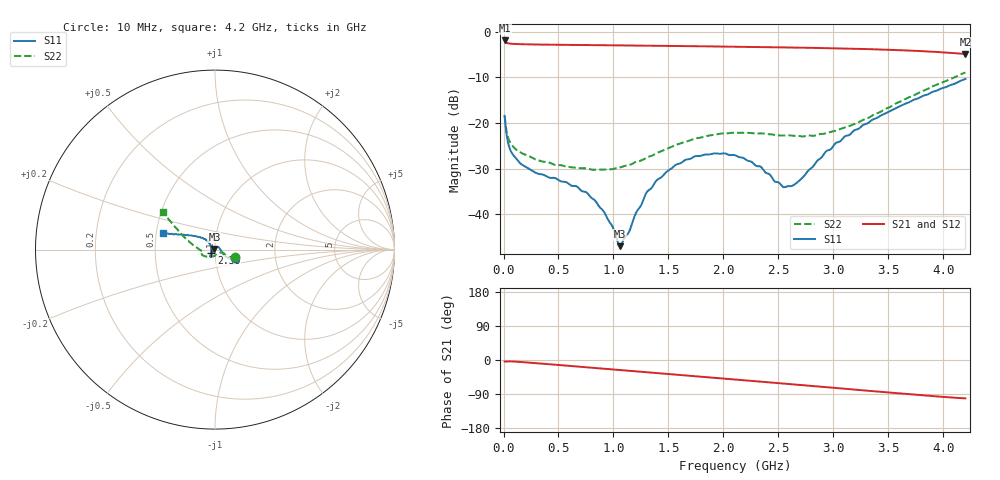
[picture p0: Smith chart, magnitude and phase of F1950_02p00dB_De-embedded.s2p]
! Integrated Device Technology
! Corporate Headquarters
! 6024 Silver Creek Valley Road
! San Jose, CA 95138  USA
! Phone:  1-408-284-8200
! Toll Free:  1-800-223-1366
! Webpage:  http://www.idt.com/
! Timing and RF Division
! 515 Groton Road, Suite 102
! Westford, MA 01886-6024
! Device:  F1950
! Description: 7-bit 0.25 dB Digital Step Attenuator
! Frequency:  150.0 -  4000.00 MHz
! Package:  4x4 mm Thin QFN Plastic Package: 24 pin
! Ports:  2 RF, 12 DC
!  Pin  1  = D0
!  Pin  2  = VDD
!  Pin  3  = Vmode
!  Pin  4  = GND
!  Pin  5  = RF1  =  Port 1
!  Pin  6  = GND
!  Pin  7  = GND
!  Pin  8  = GND
!  Pin  9  = GND
!  Pin 10  = GND
!  Pin 11  = GND
!  Pin 12  = GND
!  Pin 13  = GND
!  Pin 14  = RF2  =  Port 2
!  Pin 15  = GND
!  Pin 16  = LE
!  Pin 17  = CLK
!  Pin 18  = DATE
!  Pin 19  = D6
!  Pin 20  = D5
!  Pin 21  = D4
!  Pin 22  = D3
!  Pin 23  = D2
!  Pin 24  = D1
! State:  8
! Atten State:  2.00 dB
! Voltage:  +5.00 Volts
! Current:  Not Measured mA
! Data:  The device was measured on a the F195X evaluation board which has
!  individual transmission lines to the RF pins.  Data was collected
!  using a calibrated network analyzer.  The evaluation board was
!  de-embedded using a TRL calibration technique.
!  The reference plane is the edge of the package pin.
! Misc:  Board 2019
!  Action Tracker AT0250
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# GHz S dB R 50
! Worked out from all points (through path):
!   420 points, 10 MHz to 4.2 GHz, reference 50 ohm
!   highest |S21| = -1.93 dB at 10 MHz (marker M1); lowest = -4.9 dB at 4.2 GHz (marker M2)
!   group delay of S21, straight-line fit = 66.8 ps
!   lowest |S11| = -47.0 dB at 1.06 GHz (marker M3), VSWR 1.01, Z = 49.7 + j0.33 ohm
!   |S11| at or under -10 dB: start of sweep to end of sweep
!   |S22| runs from -30.2 to -8.9 dB; largest |S21 - S12| = 0.00089
!   S11 on the Smith chart (normalised r, x): 10 MHz: 1.24, -0.12; 2.39 GHz: 0.96, -0.04; 4.2 GHz: 0.54, +0.11
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0.01  -18.44 -22.7  -1.93 -3.8  -1.93 -3.8  -18.41 -20.7
0.06  -25.81 -27.8  -2.62 -3.6  -2.62 -3.6  -24.21 -26.0
0.16  -28.98 -12.3  -2.75 -5.3  -2.74 -5.3  -26.51 -22.1
0.3  -30.96 7.5  -2.82 -8.5  -2.82 -8.5  -28.06 -22.9
0.47  -32.05 28.0  -2.87 -12.4  -2.87 -12.4  -29.18 -25.8
0.71  -34.86 51.8  -2.93 -18.1  -2.92 -18.1  -29.89 -39.5
0.82  -36.71 61.0  -2.95 -20.8  -2.95 -20.8  -30.23 -49.6
0.91  -39.31 74.8  -2.97 -22.9  -2.97 -22.9  -30.20 -60.0
1.06  -46.95 132.3  -3.01 -26.5  -3.01 -26.5  -29.71 -81.7
1.14  -43.88 -170.3  -3.03 -28.4  -3.02 -28.4  -29.18 -92.7
1.3  -35.22 -139.2  -3.06 -32.2  -3.06 -32.2  -27.61 -112.8
1.41  -32.22 -132.3  -3.09 -34.9  -3.09 -34.9  -26.41 -123.9
1.56  -29.24 -128.3  -3.14 -38.5  -3.13 -38.5  -24.86 -135.6
1.74  -27.30 -124.8  -3.19 -42.8  -3.19 -42.8  -23.41 -146.2
2.11  -27.09 -123.7  -3.31 -51.7  -3.30 -51.7  -22.16 -159.9
2.39  -30.95 -137.7  -3.40 -58.4  -3.40 -58.4  -22.40 -165.2
2.57  -33.94 -172.2  -3.46 -62.7  -3.45 -62.7  -22.69 -168.7
2.66  -33.19 161.3  -3.49 -64.9  -3.48 -64.9  -22.78 -169.9
2.81  -29.64 136.9  -3.55 -68.6  -3.55 -68.6  -22.80 -173.4
3.1  -22.99 132.2  -3.69 -75.8  -3.68 -75.8  -21.03 179.1
3.51  -17.43 145.8  -3.97 -86.0  -3.96 -86.0  -16.56 163.2
4.2  -10.37 162.2  -4.89 -101.2  -4.89 -101.3  -8.94 144.1
